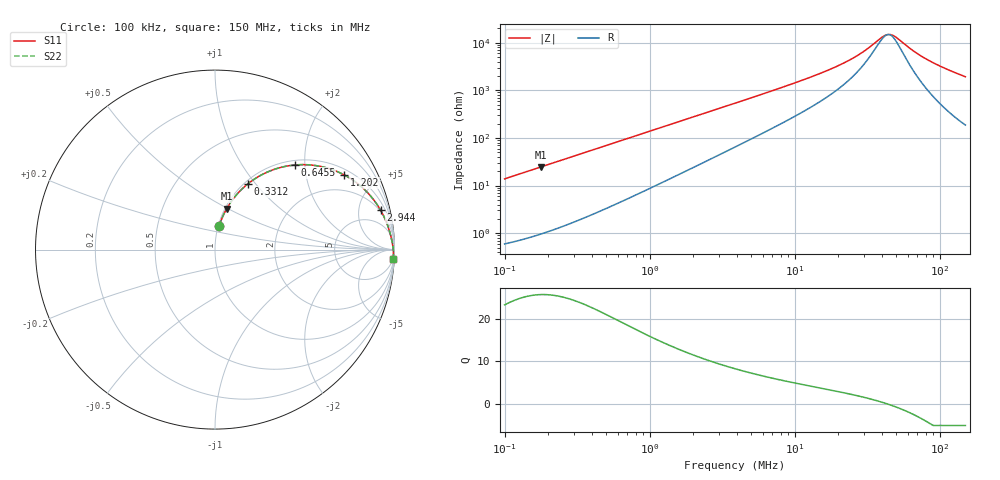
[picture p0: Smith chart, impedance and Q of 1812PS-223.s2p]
# MHz S MA R 50
!Freq  MagS11  AngS11  MagS21  AngS21  MagS12  AngS12  MagS22  AngS22
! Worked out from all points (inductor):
!   801 points, 100 kHz to 150 MHz, reference 50 ohm
!   read as one part in series: L = 22 uH near 103.7 kHz
!   highest Q = 25.6 at 177.9 kHz (marker M1), where L = 22 uH
!   self-resonance near 43.81 MHz
!   S11 on the Smith chart (normalised r, x): 100 kHz: 1.01, +0.28; 331.2 kHz: 1.04, +0.91; 645.5 kHz: 1.09, +1.78; 1.202 MHz: 1.23, +3.31; 2.944 MHz: 1.85, +8.09; 150 MHz: 5, -38
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0.1  0.1362 79.7  0.9848 -7.8  0.9848 -7.8  0.1362 79.7
0.1778759  0.2367 74.1  0.9624 -13.7  0.9624 -13.7  0.2367 74.1
0.3311959  0.4097 63.4  0.8951 -24.2  0.8951 -24.2  0.4097 63.4
0.3404045  0.4189 62.8  0.8905 -24.7  0.8905 -24.7  0.4189 62.8
0.6455104  0.6488 46.6  0.7277 -40.4  0.7277 -40.4  0.6488 46.6
0.8491936  0.7398 39.0  0.6309 -47.6  0.6309 -47.6  0.7398 39.0
1.148208  0.8213 31.1  0.5181 -55.0  0.5181 -55.0  0.8213 31.1
1.201907  0.8317 30.0  0.5013 -56.1  0.5013 -56.1  0.8317 30.0
1.83019  0.9044 20.9  0.358 -64.3  0.358 -64.3  0.9044 20.9
2.94403  0.9483 13.4  0.2332 -70.6  0.2332 -70.6  0.9483 13.4
3.872983  0.9624 10.3  0.1796 -72.8  0.1796 -72.8  0.9624 10.3
13.18381  0.9868 2.8  0.05067 -73.5  0.05067 -73.5  0.9868 2.8
18.65973  0.9894 1.8  0.03297 -70.4  0.03297 -70.4  0.9894 1.8
24.3242  0.9909 1.2  0.02222 -65.4  0.02222 -65.4  0.9909 1.2
30.29154  0.992 0.7  0.01471 -56.5  0.01471 -56.5  0.992 0.7
40.21563  0.993 0.2  0.007515 -21.8  0.007515 -21.8  0.993 0.2
44.46989  0.9933 -0.0  0.006677 4.2  0.006677 4.2  0.9933 -0.0
49.62579  0.9936 -0.2  0.007554 32.7  0.007554 32.7  0.9936 -0.2
65.88416  0.9943 -0.8  0.01489 66.9  0.01489 66.9  0.9943 -0.8
82.80067  0.9945 -1.3  0.02295 75.5  0.02295 75.5  0.9945 -1.3
109.9278  0.9945 -2.0  0.035 79.9  0.035 79.9  0.9945 -2.0
150  0.9937 -2.9  0.0516 81.5  0.0516 81.5  0.9937 -2.9
